(* Logix 5000 AddOnInstructionDefinition export Banner_TL50Pro_Param_v4; software revision 33.00; part 2 of 2 *)
(* tags used below, declared in another part *)
   TL50_Pro : Banner_TL50Pro_v4;
   Port_Data : Banner_IOL_Port_v4;
   Port : INT;   // Port Number that device is plugged into.
   Local_Control : DINT;
   Command_Being_Processed : BOOL;
   Update_Archive : BOOL;
   Index_Write_Inprocess : DINT;
   Inprocess_Index : DINT;
   SB_W_Index : DINT;
(* Banner_TL50Pro_Param_v4, continued *)

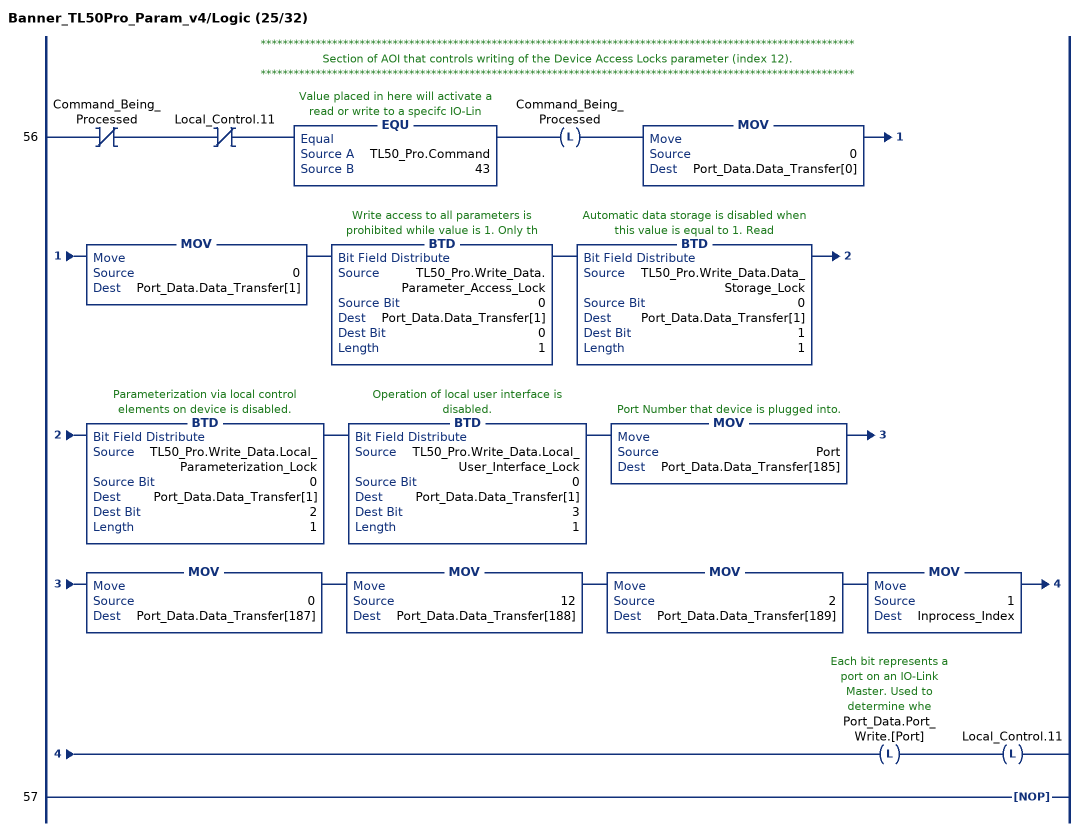
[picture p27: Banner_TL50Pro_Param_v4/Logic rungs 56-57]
   // ************************************************************************************************************
   // Section of AOI that controls writing of the Device Access Locks parameter (index 12).
   // ************************************************************************************************************
   56: XIO(Command_Being_Processed)XIO(Local_Control.11)EQU(TL50_Pro.Command,43)OTL(Command_Being_Processed)MOV(0,Port_Data.Data_Transfer[0])MOV(0,Port_Data.Data_Transfer[1])BTD(TL50_Pro.Write_Data.Parameter_Access_Lock,0,Port_Data.Data_Transfer[1],0,1)BTD(TL50_Pro.Write_Data.Data_Storage_Lock,0,Port_Data.Data_Transfer[1],1,1)BTD(TL50_Pro.Write_Data.Local_Parameterization_Lock,0,Port_Data.Data_Transfer[1],2,1)BTD(TL50_Pro.Write_Data.Local_User_Interface_Lock,0,Port_Data.Data_Transfer[1],3,1)MOV(Port,Port_Data.Data_Transfer[185])MOV(0,Port_Data.Data_Transfer[187])MOV(12,Port_Data.Data_Transfer[188])MOV(2,Port_Data.Data_Transfer[189])MOV(1,Inprocess_Index)OTL(Port_Data.Port_Write.[Port])OTL(Local_Control.11);
   57: NOP();
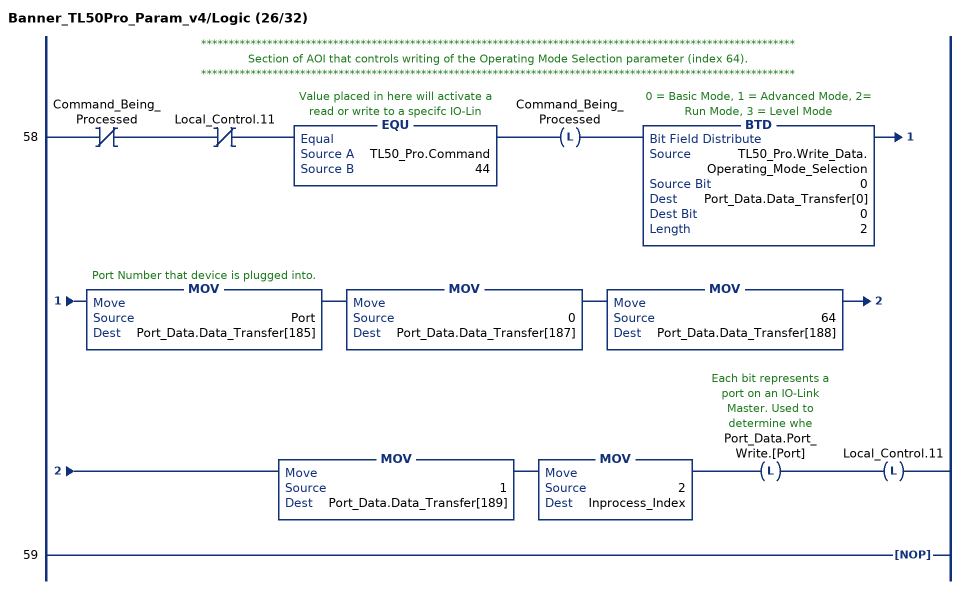
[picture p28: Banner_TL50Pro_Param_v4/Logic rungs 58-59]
   // ************************************************************************************************************
   // Section of AOI that controls writing of the Operating Mode Selection parameter (index 64).
   // ************************************************************************************************************
   58: XIO(Command_Being_Processed)XIO(Local_Control.11)EQU(TL50_Pro.Command,44)OTL(Command_Being_Processed)BTD(TL50_Pro.Write_Data.Operating_Mode_Selection,0,Port_Data.Data_Transfer[0],0,2)MOV(Port,Port_Data.Data_Transfer[185])MOV(0,Port_Data.Data_Transfer[187])MOV(64,Port_Data.Data_Transfer[188])MOV(1,Port_Data.Data_Transfer[189])MOV(2,Inprocess_Index)OTL(Port_Data.Port_Write.[Port])OTL(Local_Control.11);
   59: NOP();
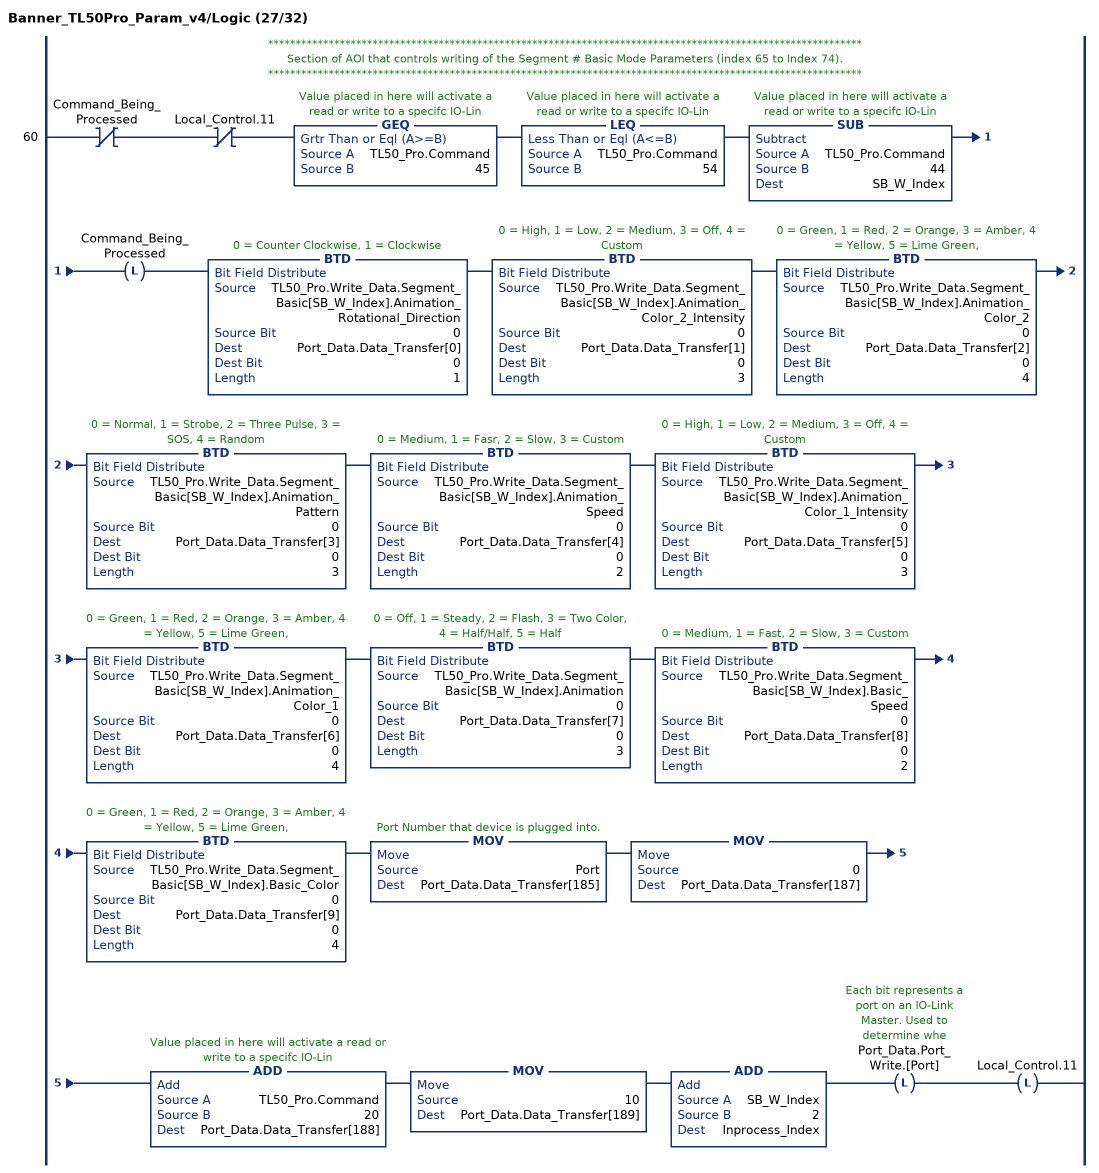
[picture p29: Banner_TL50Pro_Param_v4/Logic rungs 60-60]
   // ************************************************************************************************************
   // Section of AOI that controls writing of the Segment # Basic Mode Parameters (index 65 to Index 74).
   // ************************************************************************************************************
   60: XIO(Command_Being_Processed)XIO(Local_Control.11)GEQ(TL50_Pro.Command,45)LEQ(TL50_Pro.Command,54)SUB(TL50_Pro.Command,44,SB_W_Index)OTL(Command_Being_Processed)BTD(TL50_Pro.Write_Data.Segment_Basic[SB_W_Index].Animation_Rotational_Direction,0,Port_Data.Data_Transfer[0],0,1)BTD(TL50_Pro.Write_Data.Segment_Basic[SB_W_Index].Animation_Color_2_Intensity,0,Port_Data.Data_Transfer[1],0,3)BTD(TL50_Pro.Write_Data.Segment_Basic[SB_W_Index].Animation_Color_2,0,Port_Data.Data_Transfer[2],0,4)BTD(TL50_Pro.Write_Data.Segment_Basic[SB_W_Index].Animation_Pattern,0,Port_Data.Data_Transfer[3],0,3)BTD(TL50_Pro.Write_Data.Segment_Basic[SB_W_Index].Animation_Speed,0,Port_Data.Data_Transfer[4],0,2)BTD(TL50_Pro.Write_Data.Segment_Basic[SB_W_Index].Animation_Color_1_Intensity,0,Port_Data.Data_Transfer[5],0,3)BTD(TL50_Pro.Write_Data.Segment_Basic[SB_W_Index].Animation_Color_1,0,Port_Data.Data_Transfer[6],0,4)BTD(TL50_Pro.Write_Data.Segment_Basic[SB_W_Index].Animation,0,Port_Data.Data_Transfer[7],0,3)BTD(TL50_Pro.Write_Data.Segment_Basic[SB_W_Index].Basic_Speed,0,Port_Data.Data_Transfer[8],0,2)BTD(TL50_Pro.Write_Data.Segment_Basic[SB_W_Index].Basic_Color,0,Port_Data.Data_Transfer[9],0,4)MOV(Port,Port_Data.Data_Transfer[185])MOV(0,Port_Data.Data_Transfer[187])ADD(TL50_Pro.Command,20,Port_Data.Data_Transfer[188])MOV(10,Port_Data.Data_Transfer[189])ADD(SB_W_Index,2,Inprocess_Index)OTL(Port_Data.Port_Write.[Port])OTL(Local_Control.11);
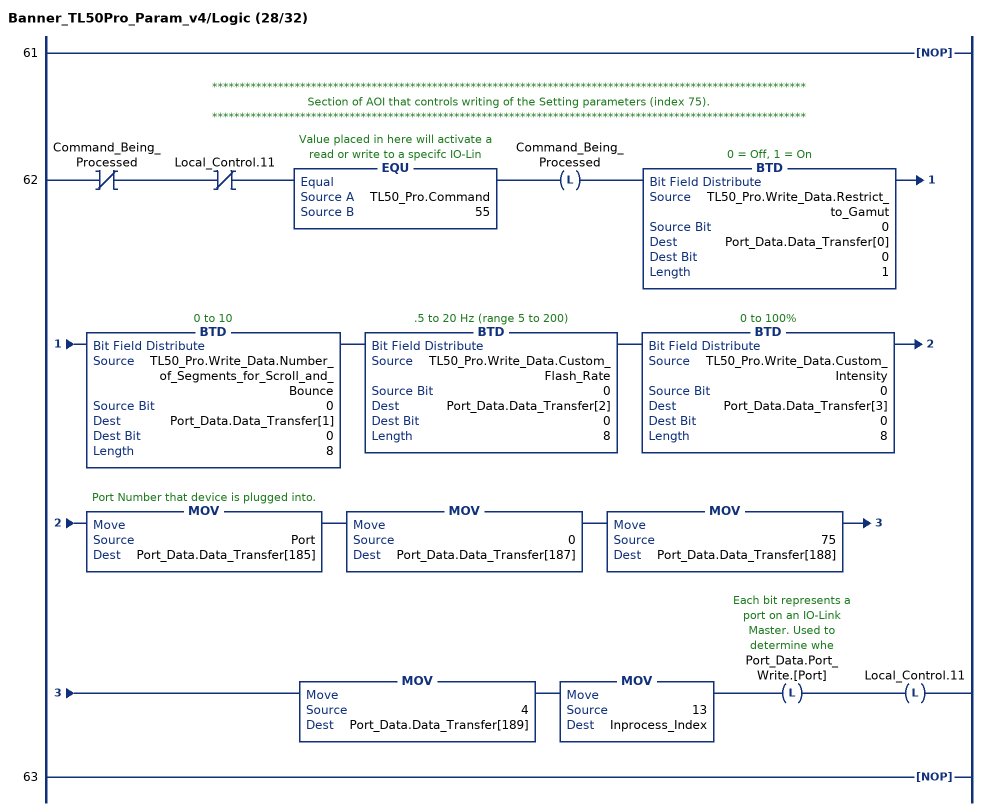
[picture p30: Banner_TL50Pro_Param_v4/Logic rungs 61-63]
   61: NOP();
   // ************************************************************************************************************
   // Section of AOI that controls writing of the Setting parameters (index 75).
   // ************************************************************************************************************
   62: XIO(Command_Being_Processed)XIO(Local_Control.11)EQU(TL50_Pro.Command,55)OTL(Command_Being_Processed)BTD(TL50_Pro.Write_Data.Restrict_to_Gamut,0,Port_Data.Data_Transfer[0],0,1)BTD(TL50_Pro.Write_Data.Number_of_Segments_for_Scroll_and_Bounce,0,Port_Data.Data_Transfer[1],0,8)BTD(TL50_Pro.Write_Data.Custom_Flash_Rate,0,Port_Data.Data_Transfer[2],0,8)BTD(TL50_Pro.Write_Data.Custom_Intensity,0,Port_Data.Data_Transfer[3],0,8)MOV(Port,Port_Data.Data_Transfer[185])MOV(0,Port_Data.Data_Transfer[187])MOV(75,Port_Data.Data_Transfer[188])MOV(4,Port_Data.Data_Transfer[189])MOV(13,Inprocess_Index)OTL(Port_Data.Port_Write.[Port])OTL(Local_Control.11);
   63: NOP();
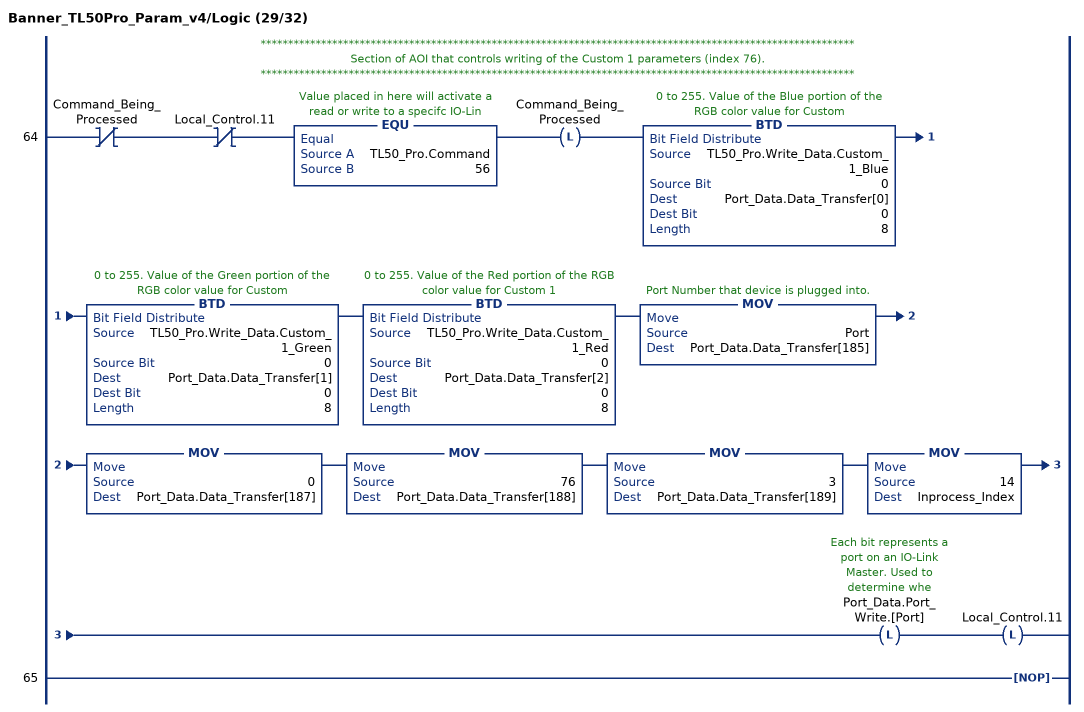
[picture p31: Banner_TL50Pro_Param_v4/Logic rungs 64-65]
   // ************************************************************************************************************
   // Section of AOI that controls writing of the Custom 1 parameters (index 76).
   // ************************************************************************************************************
   64: XIO(Command_Being_Processed)XIO(Local_Control.11)EQU(TL50_Pro.Command,56)OTL(Command_Being_Processed)BTD(TL50_Pro.Write_Data.Custom_1_Blue,0,Port_Data.Data_Transfer[0],0,8)BTD(TL50_Pro.Write_Data.Custom_1_Green,0,Port_Data.Data_Transfer[1],0,8)BTD(TL50_Pro.Write_Data.Custom_1_Red,0,Port_Data.Data_Transfer[2],0,8)MOV(Port,Port_Data.Data_Transfer[185])MOV(0,Port_Data.Data_Transfer[187])MOV(76,Port_Data.Data_Transfer[188])MOV(3,Port_Data.Data_Transfer[189])MOV(14,Inprocess_Index)OTL(Port_Data.Port_Write.[Port])OTL(Local_Control.11);
   65: NOP();
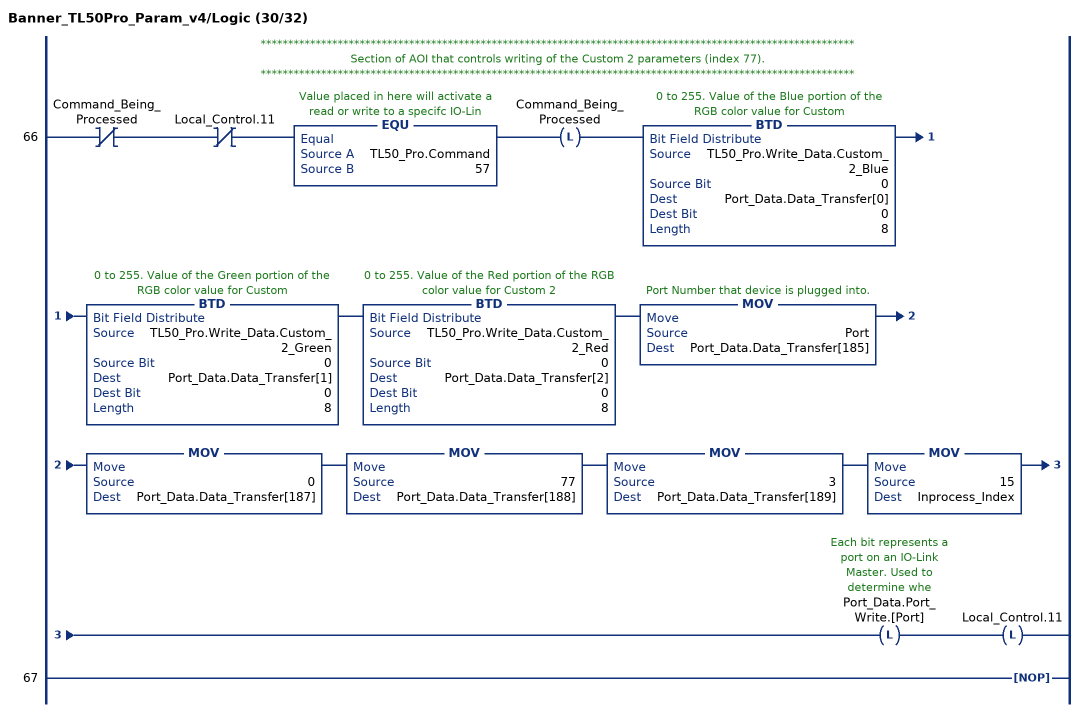
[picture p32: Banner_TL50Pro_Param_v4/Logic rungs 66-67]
   // ************************************************************************************************************
   // Section of AOI that controls writing of the Custom 2 parameters (index 77).
   // ************************************************************************************************************
   66: XIO(Command_Being_Processed)XIO(Local_Control.11)EQU(TL50_Pro.Command,57)OTL(Command_Being_Processed)BTD(TL50_Pro.Write_Data.Custom_2_Blue,0,Port_Data.Data_Transfer[0],0,8)BTD(TL50_Pro.Write_Data.Custom_2_Green,0,Port_Data.Data_Transfer[1],0,8)BTD(TL50_Pro.Write_Data.Custom_2_Red,0,Port_Data.Data_Transfer[2],0,8)MOV(Port,Port_Data.Data_Transfer[185])MOV(0,Port_Data.Data_Transfer[187])MOV(77,Port_Data.Data_Transfer[188])MOV(3,Port_Data.Data_Transfer[189])MOV(15,Inprocess_Index)OTL(Port_Data.Port_Write.[Port])OTL(Local_Control.11);
   67: NOP();
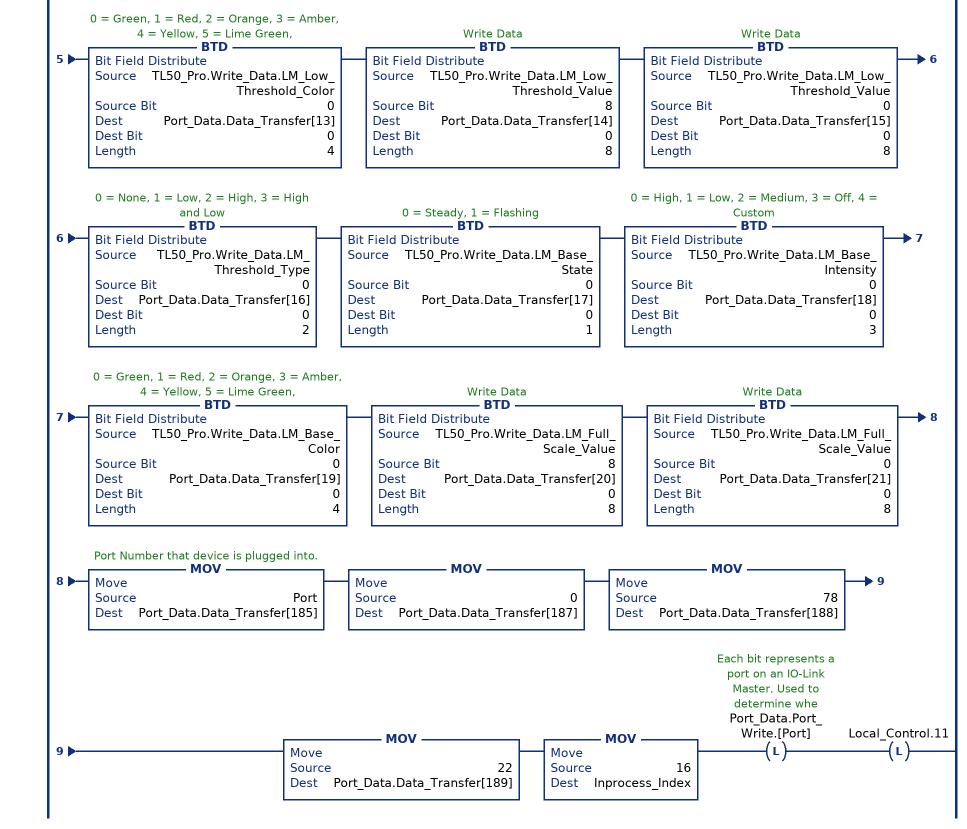
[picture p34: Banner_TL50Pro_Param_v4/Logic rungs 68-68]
   // ************************************************************************************************************
   // Section of AOI that controls writing of the LeveL Mode Configuration parameters (index 78).
   // ************************************************************************************************************
   68: XIO(Command_Being_Processed)XIO(Local_Control.11)EQU(TL50_Pro.Command,58)OTL(Command_Being_Processed)BTD(TL50_Pro.Write_Data.LM_Orientation,0,Port_Data.Data_Transfer[0],0,1)BTD(TL50_Pro.Write_Data.LM_Background_Intensity,0,Port_Data.Data_Transfer[1],0,3)BTD(TL50_Pro.Write_Data.LM_Background_Color,0,Port_Data.Data_Transfer[2],0,4)BTD(TL50_Pro.Write_Data.LM_Subsegment_Style,0,Port_Data.Data_Transfer[3],0,2)BTD(TL50_Pro.Write_Data.LM_Dominance,0,Port_Data.Data_Transfer[4],0,1)BTD(TL50_Pro.Write_Data.LM_Flash_Rate,0,Port_Data.Data_Transfer[5],0,2)BTD(TL50_Pro.Write_Data.LM_High_Threshold_State,0,Port_Data.Data_Transfer[6],0,1)BTD(TL50_Pro.Write_Data.LM_High_Threshold_Intensity,0,Port_Data.Data_Transfer[7],0,3)BTD(TL50_Pro.Write_Data.LM_High_Threshold_Color,0,Port_Data.Data_Transfer[8],0,4)BTD(TL50_Pro.Write_Data.LM_High_Threshold_Value,8,Port_Data.Data_Transfer[9],0,8)BTD(TL50_Pro.Write_Data.LM_High_Threshold_Value,0,Port_Data.Data_Transfer[10],0,8)BTD(TL50_Pro.Write_Data.LM_Low_Threshold_State,0,Port_Data.Data_Transfer[11],0,1)BTD(TL50_Pro.Write_Data.LM_Low_Threshold_Intensity,0,Port_Data.Data_Transfer[12],0,3)BTD(TL50_Pro.Write_Data.LM_Low_Threshold_Color,0,Port_Data.Data_Transfer[13],0,4)BTD(TL50_Pro.Write_Data.LM_Low_Threshold_Value,8,Port_Data.Data_Transfer[14],0,8)BTD(TL50_Pro.Write_Data.LM_Low_Threshold_Value,0,Port_Data.Data_Transfer[15],0,8)BTD(TL50_Pro.Write_Data.LM_Threshold_Type,0,Port_Data.Data_Transfer[16],0,2)BTD(TL50_Pro.Write_Data.LM_Base_State,0,Port_Data.Data_Transfer[17],0,1)BTD(TL50_Pro.Write_Data.LM_Base_Intensity,0,Port_Data.Data_Transfer[18],0,3)BTD(TL50_Pro.Write_Data.LM_Base_Color,0,Port_Data.Data_Transfer[19],0,4)BTD(TL50_Pro.Write_Data.LM_Full_Scale_Value,8,Port_Data.Data_Transfer[20],0,8)BTD(TL50_Pro.Write_Data.LM_Full_Scale_Value,0,Port_Data.Data_Transfer[21],0,8)MOV(Port,Port_Data.Data_Transfer[185])MOV(0,Port_Data.Data_Transfer[187])MOV(78,Port_Data.Data_Transfer[188])MOV(22,Port_Data.Data_Transfer[189])MOV(16,Inprocess_Index)OTL(Port_Data.Port_Write.[Port])OTL(Local_Control.11);
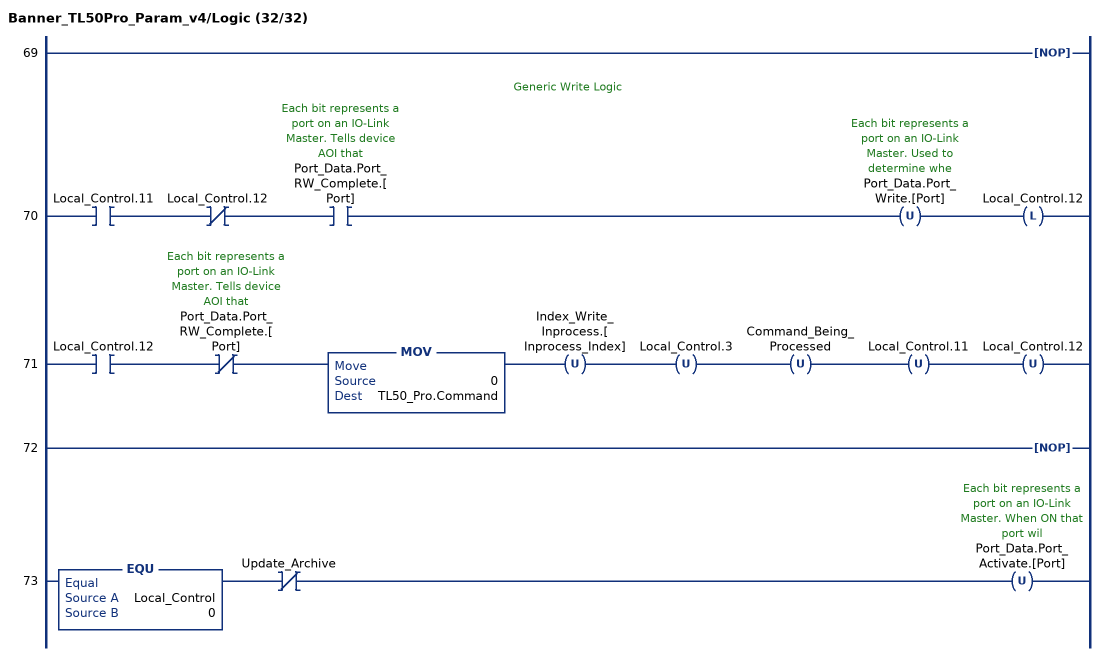
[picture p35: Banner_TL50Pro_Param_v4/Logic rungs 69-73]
   69: NOP();
   // Generic Write Logic
   70: XIC(Local_Control.11)XIO(Local_Control.12)XIC(Port_Data.Port_RW_Complete.[Port])OTU(Port_Data.Port_Write.[Port])OTL(Local_Control.12);
   71: XIC(Local_Control.12)XIO(Port_Data.Port_RW_Complete.[Port])MOV(0,TL50_Pro.Command)OTU(Index_Write_Inprocess.[Inprocess_Index])OTU(Local_Control.3)OTU(Command_Being_Processed)OTU(Local_Control.11)OTU(Local_Control.12);
   72: NOP();
   73: EQU(Local_Control,0)XIO(Update_Archive)OTU(Port_Data.Port_Activate.[Port]);
END_ROUTINE
END_ADD_ON_INSTRUCTION
